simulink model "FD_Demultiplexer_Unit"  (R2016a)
settings: Solver=ode3  StartTime=0.0  StopTime=6  FixedStep=1/5000000  RelTol=1e-3
undefined symbols (not defined in the file or in its folder): K
libraries: dsparch4 x1, commsynccomp2 x1, simulink x1

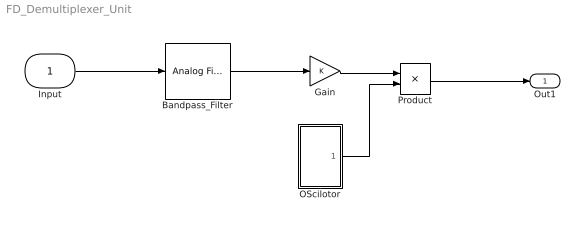
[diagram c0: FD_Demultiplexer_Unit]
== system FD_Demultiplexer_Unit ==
  Input : Inport
  Bandpass_Filter : dsparch4/Analog Filter Design  method=Butterworth  filttype=Bandpass  N=8  Wlo=589000*2*pi  Whi=689000*2*pi  Rp=2  Rs=40
  Gain : Gain  Gain=K
  OScilotor : Subsystem
  Product : Product
  Out1 : Outport
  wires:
  Input/1 -> Bandpass_Filter/1
  OScilotor/1(Output) -> Product/2
  Product/1 -> Out1/1
  Bandpass_Filter/1 -> Gain/1
  Gain/1 -> Product/1

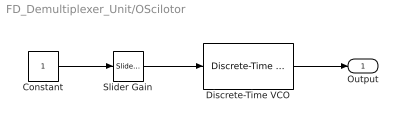
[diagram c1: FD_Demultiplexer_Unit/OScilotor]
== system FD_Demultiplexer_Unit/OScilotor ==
  Constant : Constant
  Discrete-Time VCO : commsynccomp2/Discrete-Time VCO  Ac=1  Fc=0  Kc=1000  Ph=0  ts=1/5000000
  Slider Gain : simulink/Math Operations/Slider Gain  low=139  gain=139  high=2070
  Output : Outport
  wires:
  Constant/1 -> Slider Gain/1
  Slider Gain/1 -> Discrete-Time VCO/1
  Discrete-Time VCO/1 -> Output/1
